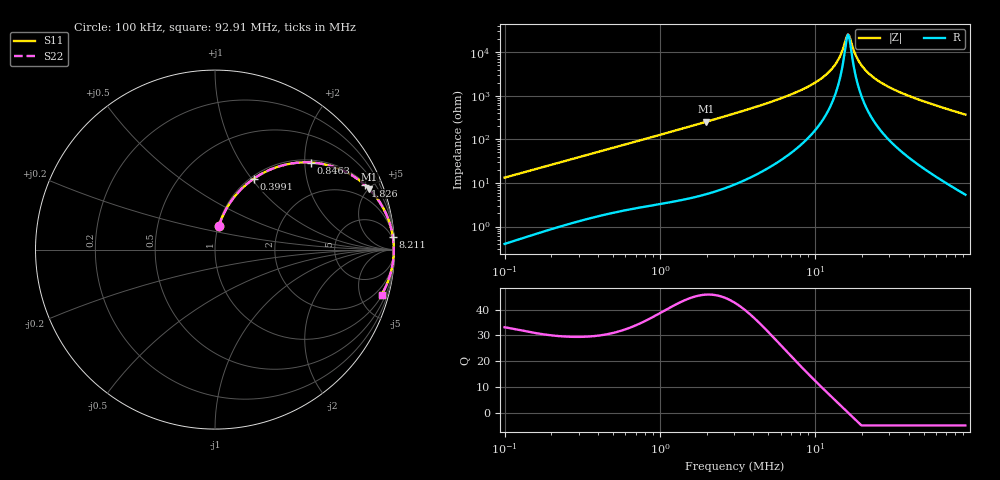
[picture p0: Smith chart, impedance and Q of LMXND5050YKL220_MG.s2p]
! LMXND5050YKL220_MG  S-PARAMETER MODEL  ( General Type )
! Model Generated by TAIYO YUDEN Corporation (https://www.yuden.co.jp/en/)
! Version 1.0
! TAIYO YUDEN Control No. 191023NI43SB-FBB
! Copyright(c) 2019 TAIYO YUDEN CO.,LTD. All Rights Reserved.
! Product Description (link to TY-COMPAS)
! https://ds.yuden.co.jp/TYCOMPAS/or/detail?pn=LMXND5050YKL220MMG&u=M
! Products Name : Inductors
! Characteristics :
!  Inductance : 22 uH , SRF(min) : 9.0 MHz , DC Resistance(max) : 0.1638 Ohm
!  Rated Current : Saturation :1500 mA , Temp Rise : 1400 mA (40 degC)
!  Case Size : 4.9 x 4.9 / 0.193 x 0.193 [mm/inch] , Thickness : 4 / 0.157 [mm/inch]
!  (Conditions: Temperature = 25 degC , DC Bias Current/Voltage = 0A / 0V)
! External Node Assignments :
!  1  o---GGG---o  2
! GND o---------o GND
! Frequency Range : 0.1MHz  -  92.907885MHz  [ 402 STEP ]
# MHz S RI R 50
! Freq[MHz].  S11 Real  S11 Imag  S21 Real  S21 Imag  S12 Real  S12 Imag  S22 Real  S22 Imag
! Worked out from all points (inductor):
!   401 points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, 100 kHz to 92.91 MHz, reference 50 ohm
!   read as one part in series: L = 21 uH near 103.5 kHz
!   highest Q = 45.8 at 1.988 MHz (marker M1), where L = 20.3 uH
!   self-resonance near 16.26 MHz
!   S11 on the Smith chart (normalised r, x): 100 kHz: 1.01, +0.27; 399.1 kHz: 1.03, +1.03; 846.3 kHz: 1.06, +2.15; 1.826 MHz: 1.10, +4.64; 8.211 MHz: 3, +27; 92.91 MHz: 1.11, -7.39
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0.1  0.0211 0.1293  0.9789 -0.1293  0.9789 -0.1293  0.0211 0.1293
0.314158  0.1503 0.3408  0.8497 -0.3408  0.8497 -0.3408  0.1503 0.3408
0.399053  0.2165 0.3954  0.7835 -0.3954  0.7835 -0.3954  0.2165 0.3954
0.846285  0.5344 0.4852  0.4656 -0.4852  0.4656 -0.4852  0.5344 0.4852
0.986956  0.6071 0.4756  0.3929 -0.4756  0.3929 -0.4756  0.6071 0.4756
1.82567  0.8379 0.3577  0.1621 -0.3577  0.1621 -0.3577  0.8379 0.3577
1.988488  0.8597 0.3366  0.1403 -0.3366  0.1403 -0.3366  0.8597 0.3366
3.100605  0.9371 0.2312  0.0629 -0.2312  0.0629 -0.2312  0.9371 0.2312
8.21096  0.9907 0.0717  0.0093 -0.0717  0.0093 -0.0717  0.9907 0.0717
9.575801  0.993 0.0541  0.00699 -0.0541  0.00699 -0.0541  0.993 0.0541
11.55571  0.9949 0.0341  0.00515 -0.0341  0.00515 -0.0341  0.9949 0.0341
13.24822  0.9956 0.0204  0.00436 -0.0204  0.00436 -0.0204  0.9956 0.0204
14.42973  0.9959 0.0119  0.00407 -0.0119  0.00407 -0.0119  0.9959 0.0119
15.71661  0.9961 0.00361  0.00392 -0.00361  0.00392 -0.00361  0.9961 0.00361
16.26294  0.9961 0.00029  0.0039 -0.00029  0.0039 -0.00029  0.9961 0.00029
16.82827  0.9961 -0.00303  0.00391 0.00303  0.00391 0.00303  0.9961 -0.00303
18.64491  0.9959 -0.013  0.00406 0.013  0.00406 0.013  0.9959 -0.013
20.65765  0.9956 -0.0232  0.00442 0.0232  0.00442 0.0232  0.9956 -0.0232
24.09141  0.9946 -0.0388  0.00538 0.0388  0.00538 0.0388  0.9946 -0.0388
30.08319  0.9921 -0.063  0.00786 0.063  0.00786 0.063  0.9921 -0.063
47.71638  0.9806 -0.1236  0.0194 0.1236  0.0194 0.1236  0.9806 -0.1236
92.90788  0.9287 -0.2502  0.0713 0.2502  0.0713 0.2502  0.9287 -0.2502
